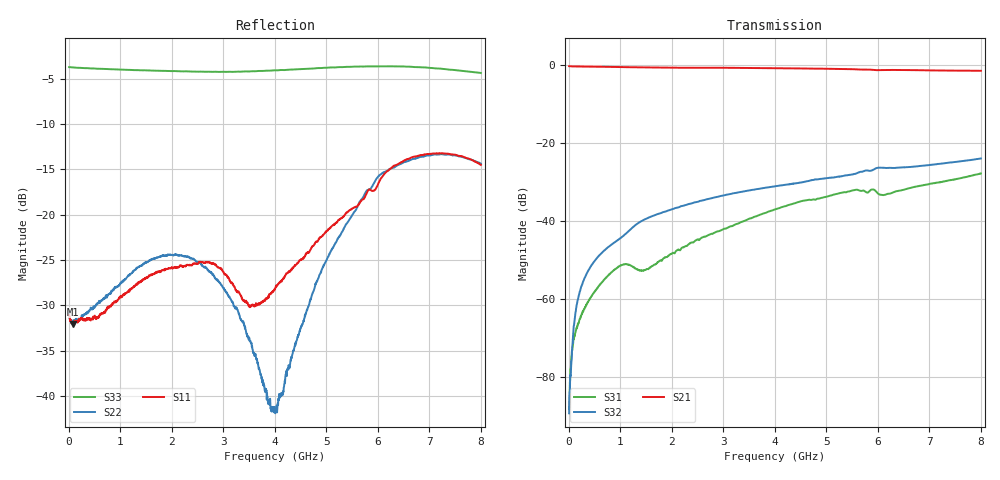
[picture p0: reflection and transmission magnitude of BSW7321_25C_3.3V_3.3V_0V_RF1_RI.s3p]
! Product: BSW7321
! Temp: 25C
! VDD: 3.300
! Control_Hi: 3.300
! Control_Lo: 0.000
! Logic State: RF1
! Port 1: RFC
! Port 2: RF1
! Port 3: RF2
! V1 = 3.30
! V2 = 0.00
! V3 = 0.00
! V4 = 0.00
# Hz S  RI  R 50
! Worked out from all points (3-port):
!   1601 points, 5 MHz to 8.005 GHz, reference 50 ohm
!   strongest paths, dB at 5 MHz, 2.005 GHz, 4.005 GHz, 6.005 GHz, 8.005 GHz:
!     S21: -0.4, -0.8, -0.9, -1.4, -1.6
!     S32: -89.2, -37.0, -31.1, -26.4, -24.0
!     S31: -88.1, -48.3, -37.0, -33.0, -27.8
!   lowest |S11| = -32.1 dB at 75 MHz (marker M1), VSWR 1.05, Z = 52.5 - j0.438 ohm
!   |S11| at or under -10 dB: start of sweep to end of sweep
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5000000  0.0277 -0.00379  0.9565 -0.0124  2.32e-05 -3.76e-05
         0.9561 -0.0123  0.029 -0.00336  3.89e-05 2.28e-06
         2.03e-05 -3.36e-05  2.92e-05 1.88e-05  -0.6506 0.00559
7.5e7  0.0246 -0.00416  0.9422 -0.1211  -0.000238 -7.78e-05
       0.9423 -0.1209  0.0252 -0.00375  -6.06e-05 0.000295
       -0.000238 -7.99e-05  -5.84e-05 0.00029  -0.6431 0.0803
9.8e8  -0.0265 -0.0228  -0.0192 -0.9318  0.00256 0.000669
       -0.0191 -0.932  -0.0239 -0.0331  0.00571 0.00144
       0.00256 0.000674  0.00571 0.00143  -0.00675 0.6309
1.94e9  -0.004 0.0504  -0.9155 -0.0121  0.00233 -0.00279
        -0.9155 -0.0121  -0.037 0.0473  0.00412 -0.0131
        0.00232 -0.00277  0.00411 -0.0131  0.6187 0.0328
2.955e9  0.0504 0.00135  0.0363 0.9112  -0.00503 -0.00569
         0.0362 0.9116  0.035 0.0217  -0.0199 -0.0065
         -0.00502 -0.00569  -0.0199 -0.00652  -0.0241 -0.6124
4.005e9  0.0297 -0.0251  0.889 -0.141  -0.0103 0.0097
         0.8892 -0.1413  -0.00351 -0.00775  -0.00824 0.0265
         -0.0102 0.00972  -0.00823 0.0265  -0.6141 0.1159
4.91e9  -0.0503 -0.0566  -0.0359 -0.8875  0.0128 0.0151
        -0.0359 -0.8874  -0.04 0.029  0.0299 0.0177
        0.0128 0.0151  0.0298 0.0177  0.0222 0.6429
5.845e9  -0.0622 0.123  -0.8639 -0.0213  0.0182 -0.016
         -0.864 -0.0214  0.0174 0.1367  0.0286 -0.0333
         0.0182 -0.0161  0.0285 -0.0334  0.6499 0.099
6.88e9  0.2126 0.0187  0.0476 0.8462  -0.0168 -0.0232
        0.048 0.8461  0.2085 -0.00956  -0.0401 -0.0315
        -0.0169 -0.0232  -0.0401 -0.0315  0.1328 -0.6345
8.005e9  -0.0665 -0.176  0.7981 -0.2439  -0.0276 0.0298
         0.7979 -0.2444  -0.0177 -0.1902  -0.0334 0.0534
         -0.0275 0.0298  -0.0334 0.0535  -0.6039 -0.00269
